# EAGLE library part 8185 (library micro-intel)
MICROCOMPUTER/PERIPHERAL DEVICE
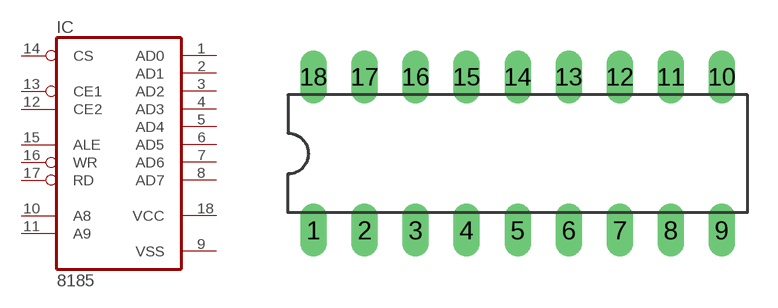
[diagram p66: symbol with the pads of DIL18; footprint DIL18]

Designator prefix IC

## 8185 (OC_FARNELL: unknown; OC_NEWARK: unknown)  [DIL18]
1  AD0
2  AD1
3  AD2
4  AD3
5  AD4
6  AD5
7  AD6
8  AD7
9  VSS  pwr
10  A8  in
11  A9  in
12  CE2  in
13  CE1  in
14  CS  in
15  ALE  in
16  WR  in
17  RD  in
18  VCC  pwr

## Footprint DIL18 (pad centres in mm)
Dual In Line Package
drill 0.813 long: 1 -10.16,-3.81; 2 -7.62,-3.81; 3 -5.08,-3.81; 4 -2.54,-3.81; 5 0,-3.81; 6 2.54,-3.81; 7 5.08,-3.81; 8 7.62,-3.81; 9 10.16,-3.81; 10 10.16,3.81; 11 7.62,3.81; 12 5.08,3.81; 13 2.54,3.81; 14 0,3.81; 15 -2.54,3.81; 16 -5.08,3.81; 17 -7.62,3.81; 18 -10.16,3.81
